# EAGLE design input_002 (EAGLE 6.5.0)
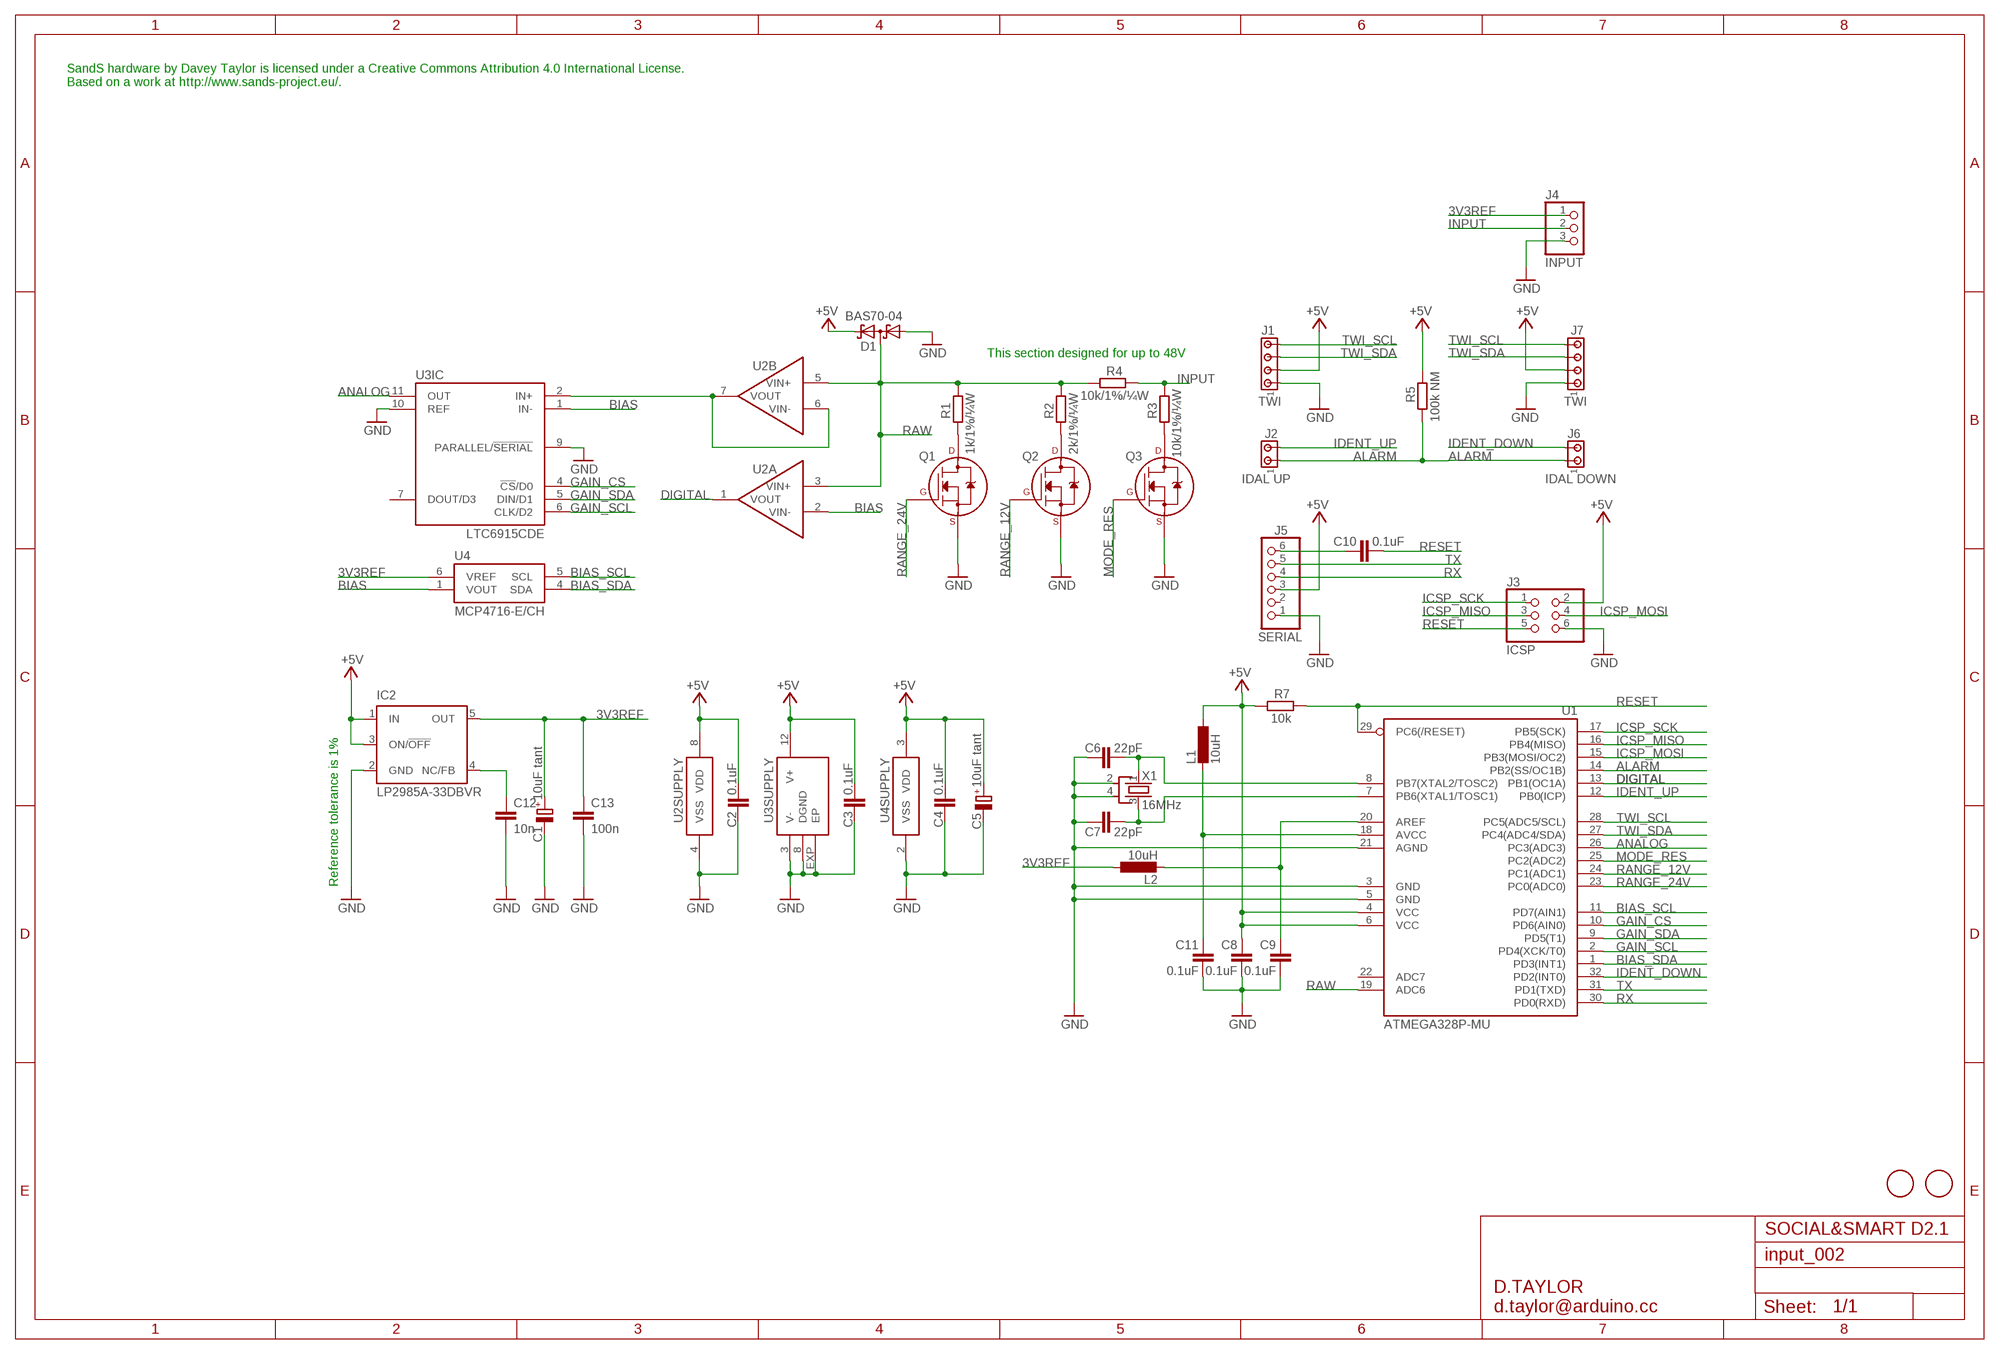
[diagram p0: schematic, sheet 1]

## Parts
C1  10uF tant  CPOL-EUSMCB  [SMC_B]
C2  0.1uF  C-EUC0603  [C0603]
C3  0.1uF  C-EUC0603  [C0603]
C4  0.1uF  C-EUC0603  [C0603]
C5  10uF tant  CPOL-EUSMCB  [SMC_B]
C6  22pF  C-EUC0603  [C0603]
C7  22pF  C-EUC0603  [C0603]
C8  0.1uF  C-EUC0603  [C0603]
C9  0.1uF  C-EUC0603  [C0603]
C10  0.1uF  C-EUC0603  [C0603]
C11  0.1uF  C-EUC0603  [C0603]
C12  10n  C-EUC0603  [C0603-ROUND]
C13  100n  C-EUC0603  [C0603-ROUND]
D1  BAS70-04  [SOT23]
IC2  LP2985A-33DBVR  LP2985-XXDBVR33  [SOT23-DBV]
J1  TWI  MTA04-100  [10X04MTA]
J2  IDAL UP  MTA02-100  [10X02MTA]
J3  ICSP  PINHD-2X3  [2X03]
J4  INPUT  MKDS_1,5/3-5,08  [MKDS1,5/3-5,08]
J5  SERIAL  PINHD-1X6  [1X06]
J6  IDAL DOWN  MTA02-100  [10X02MTA]
J7  TWI  MTA04-100  [10X04MTA]
L1  10uH  L-EUL2012C  [L2012C]
L2  10uH  L-EUL2012C  [L2012C]
Q1  2N7002_SOT23  [SOT-23]
Q2  2N7002_SOT23  [SOT-23]
Q3  2N7002_SOT23  [SOT-23]
R1  1k/1%/¼W  R-EU_R1206  [R1206]
R2  2k/1%/¼W  R-EU_R1206  [R1206]
R3  10k/1%/¼W  R-EU_R1206  [R1206]
R4  10k/1%/¼W  R-EU_R1206  [R1206]
R5  100k NM  R-EU_R0603  [R0603]
R7  10k  R-EU_R0603  [R0603]
U1  ATMEGA328P-MU  [MLF32-M1-A]
U2  MCP6402-E/SN  [SO8]
U3  LTC6915CDE  [DFN12]
U4  MCP4716-E/CH  [SOT-23-6]
U$5  FIDUCIALMOUNT  [FIDUCIA-MOUNT]
U$6  FIDUCIALMOUNT  [FIDUCIA-MOUNT]
X1  16MHz  CRYSTAL-KX7  [XTAL-3.2-2.5]

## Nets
3V3REF: C1.+ C13.1 IC2.5(OUT) J4.1 L2.1 U4.6(VREF)
+5V: C2.1 C3.1 C4.1 C5.+ C8.1 D1.2(C2) IC2.1(IN) IC2.3(ON/!OFF) J1.2 J3.2 J5.3 J7.2 L1.1 R5.2 R7.1 U1.4(VCC) U1.6(VCC) U2.8(SUPPLY:VDD) U3.12(SUPPLY:V+) U4.3(VDD)
ALARM: J2.1 J6.1 R5.1 U1.14(PB2(SS/OC1B))
ANALOG: U1.26(PC3(ADC3)) U3.11(IC:OUT)
BIAS: U2.2(A:VIN-) U3.1(IC:IN-) U4.1(VOUT)
BIAS_SCL: U1.11(PD7(AIN1)) U4.5(SCL)
BIAS_SDA: U1.1(PD3(INT1)) U4.4(SDA)
DIGITAL: U1.13(PB1(OC1A)) U2.1(A:VOUT)
GAIN_CS: U1.10(PD6(AIN0)) U3.4(IC:!CS!/D0)
GAIN_SCL: U1.2(PD4(XCK/T0)) U3.6(IC:CLK/D2)
GAIN_SDA: U1.9(PD5(T1)) U3.5(IC:DIN/D1)
GND: C1.- C2.2 C3.2 C4.2 C5.- C6.1 C7.1 C8.2 C9.2 C11.2 C12.2 C13.2 D1.1(A1) IC2.2(GND) J1.1 J3.6 J4.3 J5.1 J7.1 Q1.2(S) Q2.2(S) Q3.2(S) U1.3(GND) U1.5(GND) U1.21(AGND) U2.4(SUPPLY:VSS) U3.3(SUPPLY:V-) U3.8(SUPPLY:DGND) U3.9(IC:PARALLEL/!SERIAL) U3.10(IC:REF) U3.EXP(SUPPLY:EP) U4.2(VSS) X1.2(SH1) X1.4(SH2)
ICSP_MISO: J3.3 U1.16(PB4(MISO))
ICSP_MOSI: J3.4 U1.15(PB3(MOSI/OC2))
ICSP_SCK: J3.1 U1.17(PB5(SCK))
IDENT_DOWN: J6.2 U1.32(PD2(INT0))
IDENT_UP: J2.2 U1.12(PB0(ICP))
INPUT: J4.2 R3.2 R4.2
MODE_RES: Q3.1(G) U1.25(PC2(ADC2))
N$1: Q1.3(D) R1.1
N$2: Q2.3(D) R2.1
N$3: Q3.3(D) R3.1
N$4: C12.1 IC2.4(NC/FB)
N$5: U2.6(B:VIN-) U2.7(B:VOUT) U3.2(IC:IN+)
N$6: C6.2 U1.8(PB7(XTAL2/TOSC2)) X1.1(X1)
N$7: C7.2 U1.7(PB6(XTAL1/TOSC1)) X1.3(X2)
N$8: C11.1 L1.2 U1.18(AVCC)
N$9: C10.1 J5.6
N$10: C9.1 L2.2 U1.20(AREF)
RANGE_12V: Q2.1(G) U1.24(PC1(ADC1))
RANGE_24V: Q1.1(G) U1.23(PC0(ADC0))
RAW: D1.3(C1A2) R1.2 R2.2 R4.1 U1.19(ADC6) U2.3(A:VIN+) U2.5(B:VIN+)
RESET: C10.2 J3.5 R7.2 U1.29(PC6(/RESET))
RX: J5.4 U1.30(PD0(RXD))
TWI_SCL: J1.4 J7.4 U1.28(PC5(ADC5/SCL))
TWI_SDA: J1.3 J7.3 U1.27(PC4(ADC4/SDA))
TX: J5.5 U1.31(PD1(TXD))
Unconnected: J5.2 U1.22(ADC7) U3.7(IC:DOUT/D3)

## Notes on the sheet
- SandS hardware by Davey Taylor is licensed under a Creative Commons Attribution 4.0 International License.
  Based on a work at http://www.sands-project.eu/.
- This section designed for up to 48V
- Reference tolerance is 1%
- SOCIAL&SMART D2.1
- D.TAYLOR
  d.taylor@arduino.cc

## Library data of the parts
C1 C5 = rcl:CPOL-EU: POLARIZED CAPACITOR, European symbol
C2-C4 C6-C11 = rcl:C-EU: CAPACITOR, European symbol
C12 C13 = SmartPrj:C-EU: CAPACITOR, European symbol
D1 = diode:BAS70-04: Silicon Schottky Diodes General-purpose diode for high-speed switching
IC2 = SmartPrj:LP2985-XXDBVR: ULTRALOW-POWER 50-mA LOW-DROPOUT LINEAR REGULATORS 50-mA Low-Dropout Regulator Source: http://focus.ti.com/lit/ds/symlink/tps77001.pdf
J1 J7 = d_taylor:MTA04-100: AMP connector
J2 J6 = d_taylor:MTA02-100: AMP connector
J3 = pinhead:PINHD-2X3: PIN HEADER
J4 = d_taylor:MKDS_1,5/3-5,08: MKDSN 1,5/ 3-5,08 Printklemme Nennstrom: 13,5 A Nennspannung: 250 V Rastermaß: 5,08 mm Polzahl: 3 Anschlussart: Schraubanschluss Montage: Löten Anschlussrichtung Leiter/Platine: 0 ° Artikelnummer: 1729131 Source: http://eshop.phoenixcontact.com .. 1729131.pdf; MPN: SMKDSN1,5/3-5,08; OC_FARNELL: 1792904; OC_NEWARK: 70R0299
J5 = pinhead:PINHD-1X6: PIN HEADER
L1 L2 = rcl:L-EU: INDUCTOR, European symbol
Q1-Q3 = d_taylor:2N700*: 2N7000, 2N7002, NDS7002A N-channel enhancement mode MOSFET
R1-R5 R7 = rcl:R-EU_: RESISTOR, European symbol
U1 = d_taylor:ATMEGA*: MICROCONTROLLER 8 Kbytes FLASH 1 kbytes SRAM 512 bytes EEPROM USART 6-channel 10 bit ADC 2-channel 8 bit ADC Source: avr.lbr
U2 = d_taylor:MCP6402
U3 = d_taylor:LTC6915*DE
U4 = d_taylor:MCP47*6
U$5 U$6 = SmartPrj:FIDUCIALMOUNT
X1 = d_taylor:CRYSTAL-KX7

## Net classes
1 PWR: width 0.406 mm, clearance 0.254 mm
2 gnd: width 0.203 mm, drill 0.406 mm, clearance 0.203 mm
3 usbvcc: width 0.203 mm, drill 0.406 mm, clearance 0.203 mm

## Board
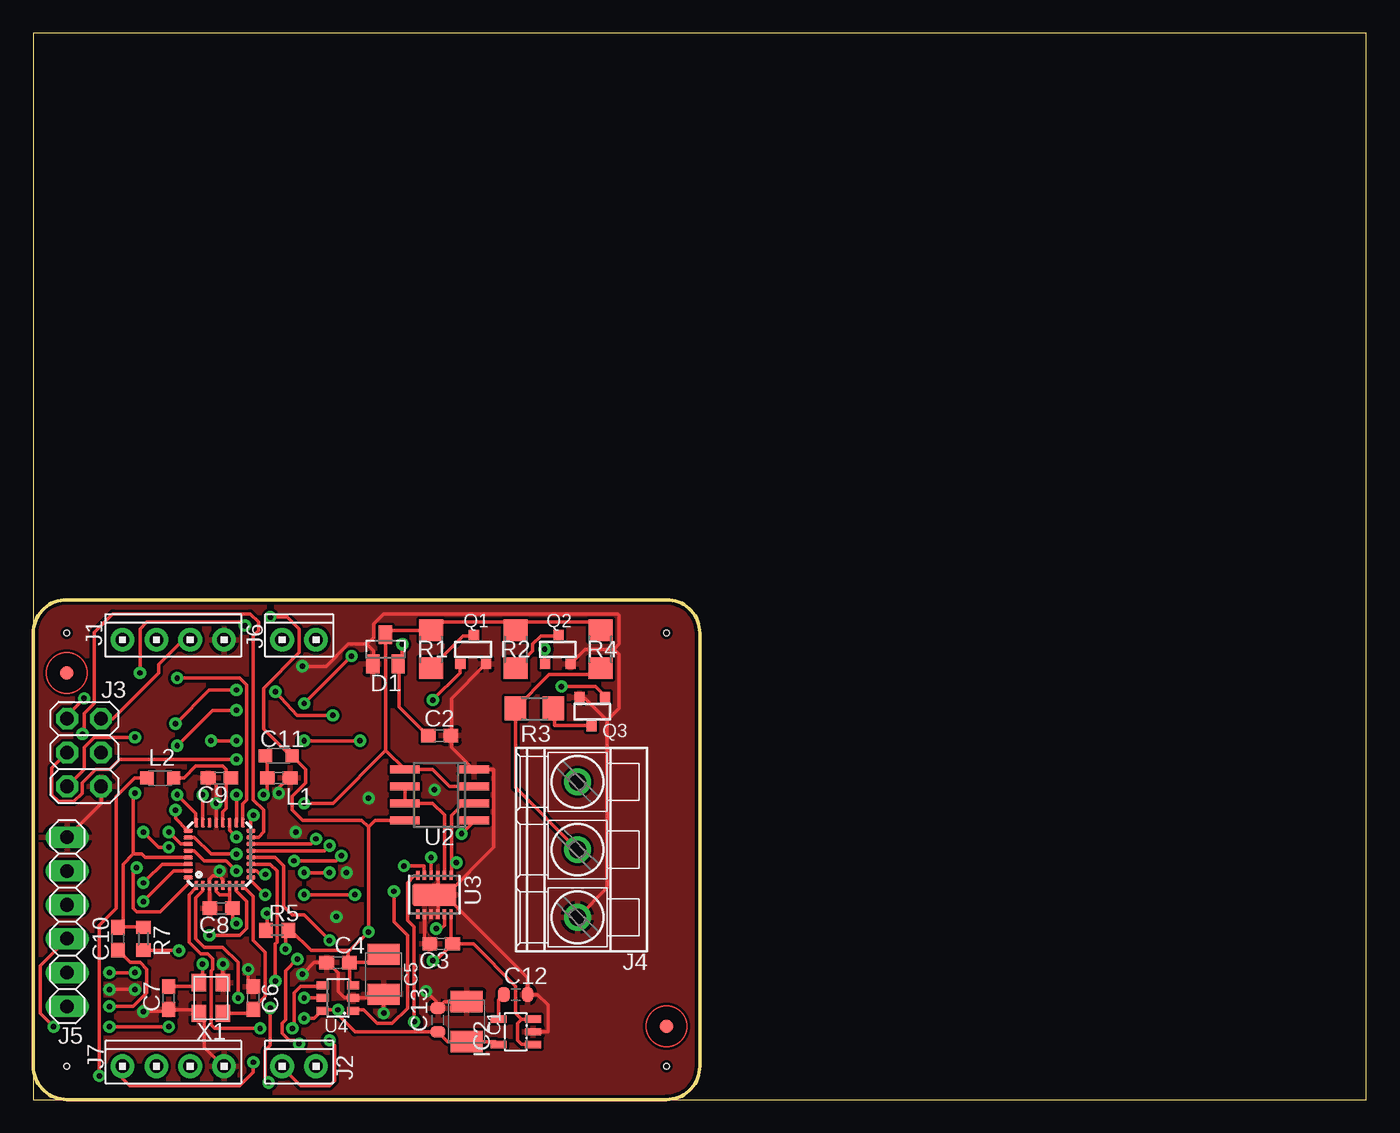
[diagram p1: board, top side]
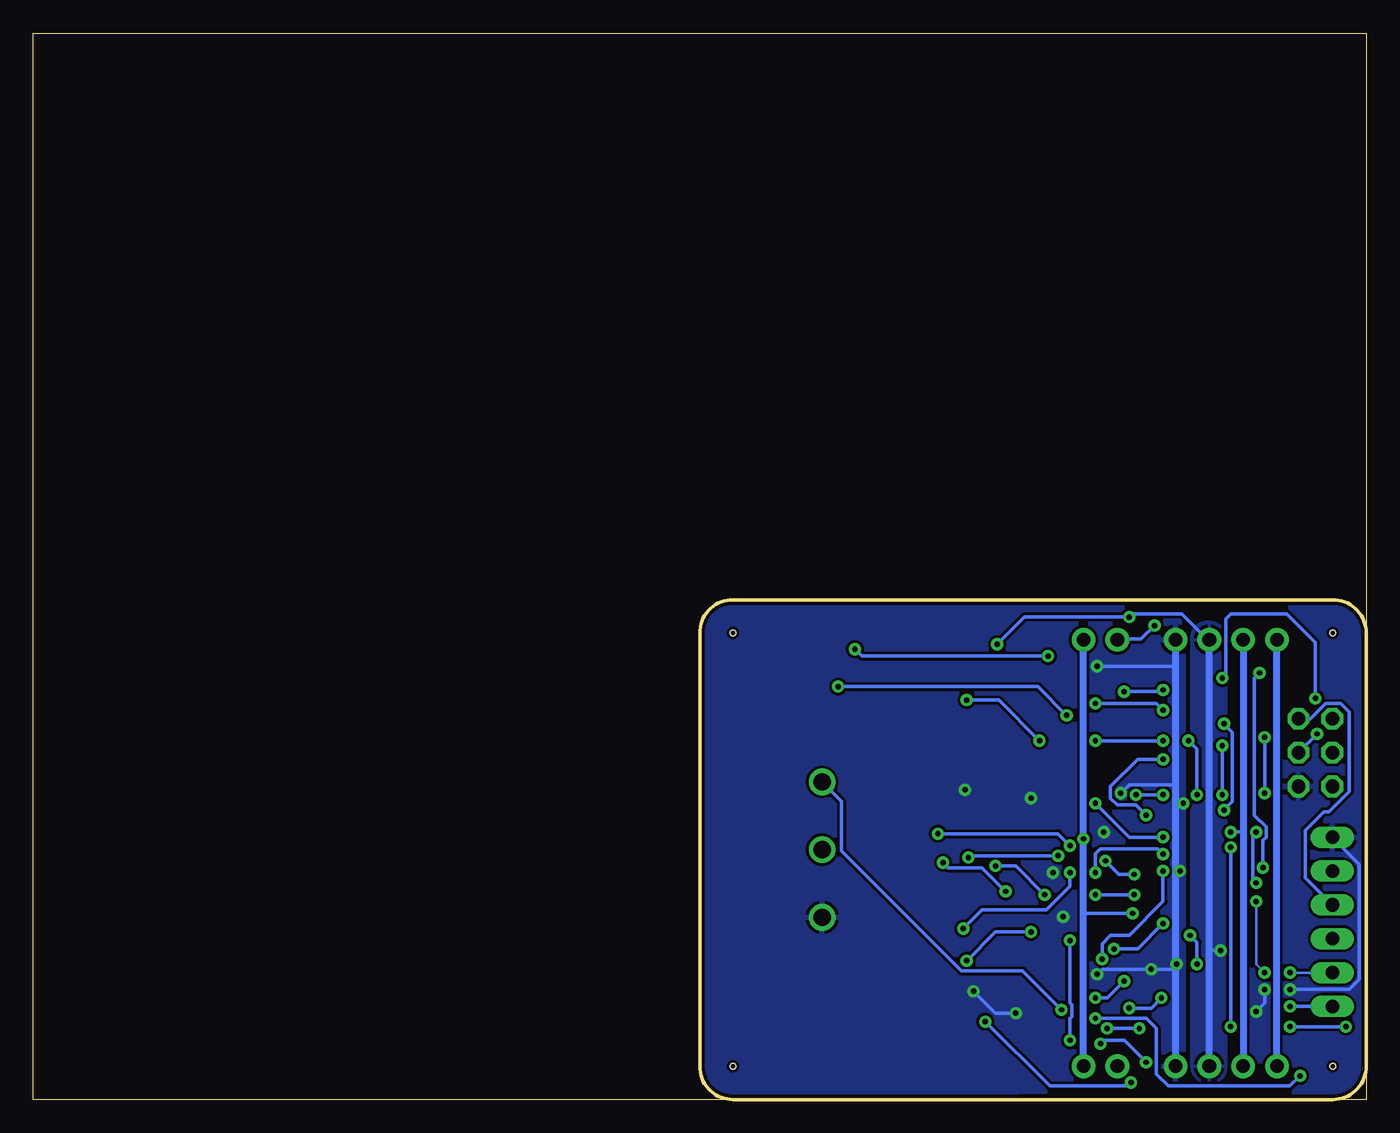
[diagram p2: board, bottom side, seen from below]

Size 100 x 80 mm. Coordinates in mm from the lower left corner, seen from the top.
Outline: 0,35 0,80 100,80 100,0 0,0 0,35
Outline: 0,35 arc-90 2.5,37.5 47.5,37.5 arc-90 50,35 50,2.5 arc-90 47.5,0 2.5,0 arc-90 0,2.5 0,35
Copper layers (1*16): Top 0.035mm / dielectric 1.5mm / Bottom 0.035mm
Design rules "smartprj-mini *": minimum track width 8mil, minimum drill 10mil, track to track 8mil, track to pad 8mil, pad to pad 0.2mm, via to via 7mil, smd to smd 4mil, copper to edge 10mil, drill to drill 8mil, minimum pad ring 12mil, minimum via ring 10mil, stop-mask expansion 2mil, vias tented up to drill 20mil, thermal gap 10mil
Holes 0.41 mm at 2.5,35 2.5,2.5 47.5,2.5 47.5,35

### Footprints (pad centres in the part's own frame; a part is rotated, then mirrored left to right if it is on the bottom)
SMC_B = smd 1.6 x 2.4: + -1.5,0; - 1.5,0
C0603 = smd 1.1 x 1: 1 -0.85,0; 2 0.85,0
C0603-ROUND = smd 0.898 x 1.1: 1 -0.889,0; 2 0.889,0
SOT23 = smd 1 x 1.4: 1 -0.95,-1.1; 2 0.95,-1.1; 3 0,1.1
SOT23-DBV = smd 0.55 x 1.2: 1 -0.95,-1.3; 2 0,-1.3; 3 0.95,-1.3; 4 0.95,1.3; 5 -0.95,1.3
10X04MTA = drill 1.016 pad 1.778: 1 3.81,0; 2 1.27,0; 3 -1.27,0; 4 -3.81,0
10X02MTA = drill 1.016 pad 1.778: 1 1.27,0; 2 -1.27,0
2X03 = drill 1.016 octagon: 1 -2.54,-1.27; 2 -2.54,1.27; 3 0,-1.27; 4 0,1.27; 5 2.54,-1.27; 6 2.54,1.27
MKDS1,5/3-5,08 = drill 1.3 pad 2: 1 -5.08,0; 2 0,0; 3 5.08,0
1X06 = drill 1.016 long: 1 -6.35,0; 2 -3.81,0; 3 -1.27,0; 4 1.27,0; 5 3.81,0; 6 6.35,0
L2012C = smd 1 x 1: 1 -1,0; 2 1,0
SOT-23 = smd 0.762 x 0.762: 1 -0.979,-1.101; 2 0.94,-1.101; 3 0.025,1.067
R1206 = smd 1.6 x 1.803: 1 -1.422,0; 2 1.422,0
R0603 = smd 1 x 1.1: 1 -0.85,0; 2 0.85,0
MLF32-M1-A = smd 0.7 x 0.3: 1 -2.35,1.75; 2 -2.35,1.25; 3 -2.35,0.75; 4 -2.35,0.25; 5 -2.35,-0.25; 6 -2.35,-0.75; 7 -2.35,-1.25; 8 -2.35,-1.75; 17 2.35,-1.75; 18 2.35,-1.25; 19 2.35,-0.75; 20 2.35,-0.25; 21 2.35,0.25; 22 2.35,0.75; 23 2.35,1.25; 24 2.35,1.75 | smd 0.3 x 0.7: 9 -1.75,-2.35; 10 -1.25,-2.35; 11 -0.75,-2.35; 12 -0.25,-2.35; 13 0.25,-2.35; 14 0.75,-2.35; 15 1.25,-2.35; 16 1.75,-2.35; 25 1.75,2.35; 26 1.25,2.35; 27 0.75,2.35; 28 0.25,2.35; 29 -0.25,2.35; 30 -0.75,2.35; 31 -1.25,2.35; 32 -1.75,2.35
SO8 = smd 0.6 x 2.2: 1 -1.905,-2.6; 2 -0.635,-2.6; 3 0.635,-2.6; 4 1.905,-2.6; 5 1.905,2.6; 6 0.635,2.6; 7 -0.635,2.6; 8 -1.905,2.6
DFN12 = smd 0.25 x 0.7: 1 -1.25,-1.45; 2 -0.75,-1.45; 3 -0.25,-1.45; 4 0.25,-1.45; 5 0.75,-1.45; 6 1.25,-1.45; 7 1.25,1.45; 8 0.75,1.45; 9 0.25,1.45; 10 -0.25,1.45; 11 -0.75,1.45; 12 -1.25,1.45 | smd 3.3 x 1.7: EXP 0,0
SOT-23-6 = smd 0.6 x 0.9: 1 -0.95,-1.15; 2 0,-1.15; 3 0.95,-1.15; 4 0.95,1.15; 5 0,1.15; 6 -0.95,1.15
FIDUCIA-MOUNT = smd 1.016 x 1.016: P$1 0,0
XTAL-3.2-2.5 = smd 1.3 x 1.1: 1 -1.15,-0.9; 2 1.15,-0.9; 3 1.15,0.9; 4 -1.15,0.9

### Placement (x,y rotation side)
C1  32.51,5.84 90 top
C2  30.48,27.3 0 top
C3  30.61,11.68 180 top
C4  22.86,10.29 180 top
C5  26.29,9.4 270 top
C6  16.51,7.62 270 top
C7  10.16,7.62 90 top
C8  14.1,14.35 180 top
C9  13.97,24.13 180 top
C10  6.35,12.06 90 top
C11  18.41,24.13 0 top
C12  36.2,7.87 0 top
C13  30.35,5.97 90 top
D1  26.42,33.78 0 top
IC2  36.2,5.08 90 top
J1  10.5,34.5 0 top
J2  19.94,2.5 0 top
J3  3.81,26.04 270 top
J4  40.83,18.75 270 top
J5  2.54,13.34 270 top
J6  19.94,34.5 0 top
J7  10.5,2.5 0 top
L1  18.41,25.78 180 top
L2  9.53,24.13 0 top
Q1  33.02,33.78 0 top
Q2  39.37,33.78 0 top
Q3  41.91,29.08 180 top
R1  29.84,33.78 90 top
R2  36.2,33.78 90 top
R3  37.59,29.34 180 top
R4  42.55,33.78 270 top
R5  18.29,12.7 0 top
R7  8.26,12.06 90 top
U1  13.97,18.41 90 top
U2  30.48,22.86 90 top
U3  30.1,15.37 180 top
U4  22.86,7.62 90 top
U$5  2.5,32 0 top
U$6  47.5,5.5 0 top
X1  13.34,7.62 90 top

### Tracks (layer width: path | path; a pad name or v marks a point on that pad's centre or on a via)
3V3REF  (via drill 0.41 pad 0.61)
  Top 0.254: v4.95,1.78 4.95,13.08 6.22,14.35 6.22,22.73 7.62,24.13 8.51,24.13 L2.1 | v20.32,6.1 21.08,6.1 21.59,6.6 U4.6 21.72,6.73 v22.86,6.73 22.86,6.35 24.13,5.08 C13.1 31.09,4.34 C1.+ 34.68,4.34 IC2.5 | 40.89,23.75 J4.1
  Bottom 0.254: v22.86,6.73 25.78,9.65 30.35,9.65 39.37,18.67 39.37,22.35 40.77,23.75 J4.1 | v4.95,1.78 5.71,1.02 14.86,1.02 15.75,1.91 15.75,5.33 16.51,6.1 16.64,6.1 v20.32,6.1
+5V  (via drill 0.41 pad 0.61)
  Top 0.254: 31.11,11.68 C3.1 | 25.15,20.45 25.65,20.95 27.81,20.95 U2.8 | 25.15,20.45 24.64,20.95 24.26,20.95 20.19,20.95 19.43,21.72 19.43,22.73 20.45,23.75 20.45,24.77 19.43,25.78 L1.1 19.3,25.78 17.27,27.81 17.27,30.86 19.94,33.53 19.94,35.31 19.05,36.2 v17.78,36.2 | 14.73,15.37 13.97,15.37 13.72,15.62 13.72,16 U1.4 | 14.73,15.37 14.73,16 U1.6 | 14.73,15.37 14.73,14.35 C8.1 14.95,13.5 v15.24,13.21 | U4.3 24,8.64 23.75,8.89 23.75,10.29 C4.1 | 23.62,11.18 20.83,11.18 19.3,12.7 R5.2 18.92,12.32 v18.92,11.3 | 23.62,11.18 23.62,10.29 C4.1 | 25.15,20.45 v25.15,12.57 23.75,11.18 23.62,11.18 | C2.1 29.59,27.3 27.43,29.46 27.43,32.64 D1.2 27.43,32.77 27.69,33.02 v27.69,34.16 | v10.92,11.18 8.26,11.18 R7.1 | J3.2 5.97,28.57 9.4,32 9.4,32.64 11.18,34.42 J1.2 | v29.97,10.41 30.23,10.45 C3.1 | U3.12 31.35,12.08 C3.1 | IC2.3 36.64,6.03 | 36.64,6.03 36.32,5.71 36.32,4.45 36.64,4.13 IC2.1 | C5.+ 25.68,10.29 C4.1 | 36.64,6.03 36.2,6.48 36.2,8.51 33.02,11.68 C3.1
  Bottom 0.254: v18.92,11.3 17.14,11.3 v15.24,13.21 | v29.97,10.41 27.81,12.57 v25.15,12.57 | v10.92,11.18 11.68,11.18 11.77,11.18 | J5.3 4.57,16.64 4.57,20.19 3.3,21.46 3.17,21.59 2.79,21.59 1.27,23.11 1.27,29.08 1.91,29.72 3.05,29.72 4.19,28.57 J3.2 | v27.69,34.16 25.65,36.2 v17.78,36.2 17.53,36.45 13.84,36.45 11.94,34.54 J1.2
  Bottom 0.508: J7.2 11.77,11.18 J1.2
  pour Bottom: 13.08,34.67 arc90 11.94,35.81 11.81,35.81 arc90 10.54,34.54 10.54,2.54 10.54,2.41 arc90 11.68,1.27 11.81,1.27 arc90 13.08,2.54
ALARM  (via drill 0.41 pad 0.61)
  Top 0.254: v21.21,19.56 20.83,19.18 16.38,19.18 U1.14 | v17.53,13.97 17.53,12.7 R5.1
  Bottom 0.254: 21.21,13.97 v17.53,13.97
  Bottom 0.508: J2.1 21.21,13.97 v21.21,19.56 J6.1
ANALOG  (via drill 0.41 pad 0.61)
  Top 0.254: v20.32,17.02 v22.23,17.02 | v15.24,18.41 13.34,18.41 12.09,19.66 U1.26 | U3.11 30.85,13.07 30.61,12.83 v30.23,12.83
  Bottom 0.254: v30.23,12.83 28.83,14.22 24,14.22 22.23,16 v22.23,17.02 | v20.32,17.02 20.32,18.41 19.94,18.8 15.62,18.8 v15.24,18.41
BIAS  (via drill 0.41 pad 0.61)
  Top 0.254: 31.37,17.78 31.37,21.34 32.26,22.23 33.02,22.23 U2.2 | 31.37,17.78 31.37,16.89 U3.1 | v27.05,15.62 27.05,13.34 28.07,12.32 28.07,6.86 26.92,5.71 25.78,5.71 24.77,6.73 24.13,6.73 U4.1 | 31.37,17.78 v31.75,17.78
  Bottom 0.254: v27.05,15.62 28.83,17.4 31.37,17.4 v31.75,17.78
BIAS_SCL  (via drill 0.41 pad 0.61)
  Top 0.254: v18.16,8.89 18.16,11.68 18.29,11.81 18.29,13.34 18.29,13.59 18.29,17.14 17.78,17.65 16.38,17.65 U1.11 | v20.32,7.62 21.59,7.62 U4.5
  Bottom 0.254: v18.16,8.89 19.43,7.62 v20.32,7.62
BIAS_SDA  (via drill 0.41 pad 0.61)
  Top 0.254: v17.02,5.33 13.59,5.33 13.34,5.59 13.34,9.65 13.46,9.78 13.46,10.54 13.08,10.92 12.57,10.92 11.68,11.81 11.68,15.37 12.19,15.88 12.22,16.03 U1.1 | v19.43,5.33 19.56,5.46 19.56,8 20.07,8.51 21.59,8.51 U4.4
  Bottom 0.254: v19.43,5.33 v17.02,5.33
DIGITAL  (via drill 0.41 pad 0.61)
  Top 0.254: v22.23,19.05 21.84,18.67 16.38,18.67 U1.13 | v32.13,19.94 33.02,20.83 33.02,20.95 U2.1
  Bottom 0.254: v22.23,19.05 23.11,19.94 v32.13,19.94
GAIN_CS  (via drill 0.41 pad 0.61)
  Top 0.254: v29.84,18.16 29.84,16.89 U3.4 | v23.11,18.29 22.73,17.91 v19.56,17.91 | v17.4,16.89 17.02,16.89 16.76,17.14 16.38,17.14 U1.10
  Bottom 0.254: v29.84,18.16 29.72,18.29 v23.11,18.29 | v19.56,17.91 18.54,16.89 v17.4,16.89
GAIN_SCL  (via drill 0.41 pad 0.61)
  Top 0.254: v15.37,7.62 15.37,10.29 14.22,11.43 12.83,11.43 12.19,12.06 12.19,15.11 12.72,15.64 U1.2 | v17.78,6.86 17.78,4.06 17.4,3.68 17.4,1.52 v17.65,1.27 | v28.57,5.84 28.57,9.53 28.57,9.78 28.57,12.95 28.07,13.46 28.07,16.26 28.57,16.76 28.83,16.76 U3.6
  Bottom 0.254: v15.37,7.62 16.13,6.86 v17.78,6.86 | v17.65,1.27 17.91,1.02 23.75,1.02 v28.57,5.84
GAIN_SDA  (via drill 0.41 pad 0.61)
  Top 0.254: v17.4,15.37 16.38,16.38 16.38,16.64 U1.9 | v24.13,15.37 v20.32,15.37 | v27.81,17.53 29.34,17.53 29.34,16.89 U3.5
  Bottom 0.254: v20.32,15.37 v17.4,15.37 | v24.13,15.37 26.29,17.53 v27.81,17.53
GND  (via drill 0.41, 0.41 pad 0.61)
  Top 0.203: 29.72,11.81 C3.2 | 31.37,27.3 C2.2 | 30.35,15.37 U3.EXP
  Top 0.254: J5.1 5.08,22.23 J3.6 | 13.21,14.48 C8.2 13.22,14.45 U1.3 13.21,16.13 13.21,16.51 13.46,16.76 13.97,16.76 | 13.97,16.76 14.22,16.51 14.22,16.13 U1.5 | U1.21 13.72,20.83 v13.72,22.23 13.72,23.62 13.21,24.13 C9.2 | v16.13,9.78 16.13,8.89 16.51,8.51 C6.1 | v18.41,22.99 18.41,23.37 19.18,24.13 C11.2 | v14.22,10.16 14.22,8.89 X1.2 | J7.1 14.22,2.54 12.83,3.94 12.83,5.97 12.45,6.35 X1.4 12.32,6.48 12.32,6.73 10.16,6.73 C7.1 10.16,6.6 v8.26,6.6 | v13.97,17.14 13.97,16.76 | v20.19,9.4 21.08,10.29 21.97,10.29 C4.2 22.1,10.29 22.86,9.53 22.86,8.13 23.37,7.62 U4.2 26.01,7.62 C5.- v26.29,6.48 | v7.62,8.26 v5.71,8.26 | 30.35,15.37 30.35,15.88 | 30.35,15.88 30.35,16.76 U3.3 | 29.72,11.81 C3.2 29.35,11.78 U3.8 U3.9 U3.10 30.35,13.97 30.35,15.11 U3.EXP | 31.37,27.3 31.37,30.1 33.91,32.64 Q1.2 | 31.37,27.3 31.37,26.42 33.02,24.77 U2.4 33.15,24.77 34.54,24.77 34.54,18.92 30.99,15.37 30.35,15.37 | 31.37,27.3 C2.2 | 30.35,15.88 32.77,13.46 37.08,9.14 C12.2 37.85,7.87 38.61,7.11 38.61,5.08 IC2.2 | 30.35,15.88 U3.EXP | 30.35,15.37 U3.EXP | 43.05,28.45 43.94,29.34 43.94,32.77 43.94,33.4 43.56,33.78 | 43.05,28.45 41.4,30.1 41.02,30.1 Q3.2 | Q2.2 40.39,32.77 41.4,33.78 43.43,33.78 43.56,33.78 | 25.02,34.16 25.53,34.67 25.53,35.69 26.29,36.45 43.81,36.45 43.94,36.32 43.94,34.16 43.56,33.78 | 25.02,34.16 25.53,33.66 25.53,32.77 D1.1 | 43.05,28.45 43.05,15.88 40.89,13.72 J4.3 | v20.19,32.51 21.97,32.51 23.62,34.16 25.02,34.16 | C1.- 30.84,7.34 C13.2 30.23,6.99 30.23,7.37 v29.46,8.13
  Bottom 0.254: 14.31,9.78 14.48,9.78 v16.13,9.78 19.81,9.78 v20.19,9.4 | v18.41,22.99 17.78,23.62 14.48,23.62 14.31,23.62 | v14.22,10.16 14.31,10.16 | v13.72,22.23 14.22,22.23 14.31,22.23 | v13.97,17.14 14.22,17.14 14.31,17.14 | J5.1 0.51,17.65 0.51,9.02 1.27,8.26 v5.71,8.26 | v7.62,8.26 7.62,7.24 v8.26,6.6 | v20.19,32.51 14.48,32.51 14.31,32.51 | v26.29,6.48 27.81,6.48 v29.46,8.13
  Bottom 0.508: J1.1 14.31,32.51 14.31,23.62 14.31,22.23 14.31,17.14 14.31,10.16 14.31,9.78 J7.1
  other vias: 19.68,20.07 22.73,13.72 25.15,22.61 30.1,23.24 23.5,17.02
  pour Top: 0.5,35 arc-90 2.5,37 47.5,37 arc-90 49.5,35 49.5,2.5 arc-90 47.5,0.5 2.5,0.5 arc-90 0.5,2.5
  pour Bottom: 0.5,35 arc-90 2.5,37 47.5,37 arc-90 49.5,35 49.5,2.5 arc-90 47.5,0.5 15.49,0.64 arc-90 13.72,2.41 13.72,34.42 arc90 11.81,36.45 arc90 9.91,34.54 9.91,2.54 arc-90 7.87,0.5 2.5,0.5 arc-90 0.5,2.5
ICSP_MISO  (via drill 0.41 pad 0.61)
  Top 0.254: v15.24,25.53 6.48,25.53 5.71,24.77 5.33,24.77 4.7,24.77 3.68,23.75 3.68,22.99 3.05,22.35 1.91,22.35 1.4,22.86 1.4,24.89 J3.3 | U1.16 16.32,21.15 v16.51,21.34
  Bottom 0.254: v16.51,21.34 17.27,22.1 18.67,22.1 19.18,22.61 19.18,23.5 17.14,25.53 v15.24,25.53
ICSP_MOSI  (via drill 0.41 pad 0.61)
  Top 0.254: v3.68,27.43 3.81,27.56 3.81,28.96 4.57,29.72 4.57,35.05 5.97,36.45 16.26,36.45 16.89,35.81 16.89,35.18 16.51,34.8 16.51,22.48 17.27,21.72 17.27,20.07 16.89,19.68 16.38,19.68 U1.15
  Bottom 0.254: J3.4 v3.68,27.43
ICSP_SCK  (via drill 0.41 pad 0.61)
  Top 0.254: v10.79,31.62 15.49,31.62 16,31.11 16,22.48 15.72,22.2 U1.17 | v3.81,30.1 2.54,28.83 J3.1
  Bottom 0.254: v10.79,31.62 10.54,31.88 10.54,32 10.54,35.94 10.54,36.07 10.16,36.45 5.97,36.45 3.81,34.29 v3.81,30.1
IDENT_DOWN  (via drill 0.41 pad 0.61)
  Top 0.254: v7.75,17.4 7.49,17.14 7.49,14.35 7.75,14.1 9.02,14.1 9.53,14.1 11.62,16.19 U1.32 | v8,32 8,32.77 8,35.31 8.51,35.81 15.62,35.81 v15.88,35.56
  Bottom 0.254: v7.75,17.4 7.75,19.43 7.49,19.68 7.49,20.45 8.38,21.34 8.38,31.62 v8,32 | v15.88,35.56 16.89,34.54 18.67,34.54 J6.2
IDENT_UP  (via drill 0.41 pad 0.61)
  Top 0.203: 18.67,2.41 J2.2
  Top 0.254: v22.23,11.94 20.32,13.84 19.43,13.84 18.8,14.48 18.8,17.53 18.16,18.16 16.38,18.16 U1.12 | v22.23,4.45 22.61,4.06 22.61,1.4 22.23,1.02 20.57,1.02 20.07,1.02 18.67,2.41
  Bottom 0.254: v22.23,11.94 22.23,7.24 22.1,7.11 22.1,6.22 22.23,6.1 v22.23,4.45
INPUT
  Top 0.254: J4.2 36.17,23.41 R3.2 38.71,31.88 41.4,31.88 41.94,31.88 R4.2
MODE_RES  (via drill 0.41 pad 0.61)
  Top 0.254: v10.67,21.72 10.67,21.08 11.56,20.19 U1.25 | v10.67,28.19 13.21,30.73 v15.24,30.73 | v18.16,30.61 19.81,28.83 v22.48,28.83 | v39.62,30.99 42.16,30.99 42.93,30.23 42.93,30.1 Q3.1
  Bottom 0.254: v10.67,21.72 10.03,22.35 10.03,27.56 v10.67,28.19 | v15.24,30.73 15.49,30.61 v18.16,30.61 | v22.48,28.83 24.64,30.99 39.12,30.99 v39.62,30.99
N$1
  Top 0.254: Q1.3 33.02,34.8 32.26,34.8 29.84,32.38 R1.1
N$2
  Top 0.254: Q2.3 39.37,34.8 38.1,34.8 37.47,34.16 37.47,33.66 36.2,32.38 R2.1
N$3
  Top 0.254: Q3.3 41.78,28.07 39.12,28.07 39.12,29.34 R3.1
N$4
  Top 0.254: 35.31,5.97 35.24,6.03 IC2.4 34.9,7.46 C12.1
N$5
  Top 0.254: U2.6 U2.7 29.97,22.23 30.85,21.35 U3.2
N$6
  Top 0.254: X1.1 14.35,6.48 16.51,6.48 16.51,6.73 C6.2 16.51,6.86 17.4,7.75 17.4,9.91 17.4,11.05 16.51,11.94 16.51,15.24 15.72,16.03 U1.8
N$7  (via drill 0.41, 0.41 pad 0.61)
  Top 0.254: v12.7,10.16 12.7,9.14 X1.3 12.32,8.76 12.32,8.51 10.16,8.51 C7.2 | 15.24,16.13 U1.7 15.22,15.64 16,14.86 16,12.83 15.49,12.32 13.34,12.32 v13.21,12.32
  Bottom 0.254: v12.7,10.16 12.7,11.81 v13.21,12.32
N$8  (via drill 0.41 pad 0.61)
  Top 0.203: 17.53,24.13 C11.1
  Top 0.254: v15.24,22.86 15.24,20.83 U1.18 | v17.27,22.86 17.53,23.11 17.53,24.13 | 17.53,24.13 17.53,25.78 L1.2 | 17.53,24.13 C11.1
  Bottom 0.254: v17.27,22.86 v15.24,22.86
N$9  (via drill 0.41 pad 0.61)
  Top 0.254: v5.71,6.99 5.84,6.99 7.49,6.99 8.51,8 8.51,9.78 8,10.29 7.49,10.29 7.28,10.29 C10.1 6.35,11.3
  Bottom 0.254: v5.71,6.99 5.46,6.99 J5.6
N$10
  Top 0.254: U1.20 14.22,20.83 14.22,21.59 14.48,21.84 14.48,23.88 14.73,24.13 C9.1 14.48,24 14.48,24.77 14.22,25.02 12.19,25.02 11.3,24.13 10.54,24.13 L2.2
RANGE_12V  (via drill 0.41 pad 0.61)
  Top 0.254: v10.79,22.86 11.43,22.23 12.19,21.46 12.19,20.83 U1.24 | v10.79,26.54 13.46,29.21 v15.24,29.21 | v23.88,33.27 v20.32,29.72 | v38.35,33.78 38.35,33.66 38.35,32.77 Q2.1
  Bottom 0.254: v10.79,26.54 v10.79,22.86 | v15.24,29.21 15.75,29.72 v20.32,29.72 | v23.88,33.27 37.85,33.27 v38.35,33.78
RANGE_24V  (via drill 0.41 pad 0.61)
  Top 0.254: v15.24,26.92 v13.34,26.92 | v24.51,26.92 v20.32,26.92 | v29.97,29.97 32,32 32,32.38 32,32.64 Q1.1 | U1.23 12.72,22.84 v12.7,22.86
  Bottom 0.254: v12.7,22.86 12.7,26.29 v13.34,26.92 | v15.24,26.92 15.62,26.92 v20.32,26.92 | v24.51,26.92 27.56,29.97 v29.97,29.97
RAW  (via drill 0.41)
  Top 0.254: R4.1 41.94,35.81 39.37,35.81 36.8,35.81 R2.2 35.59,35.81 33.02,35.81 30.45,35.81 R1.2 26.74,35.2 D1.3 26.42,26.23 26.45,26.2 | 26.45,26.2 U2.5 29.97,24.77 31.24,23.5 U2.3 | U1.19 14.72,20.2 v15.24,19.68 | v20.32,22.23 22.48,22.23 26.45,26.2
  Bottom 0.254: v15.24,19.68 17.78,19.68 v20.32,22.23
RESET  (via drill 0.41 pad 0.51, 0.41 pad 0.61)
  Top 0.254: 7.49,18.41 8.13,18.41 8.38,18.16 11.56,18.16 U1.29 | 7.49,18.41 6.73,17.65 6.73,13.34 6.35,12.95 C10.2 6.48,12.95 8.26,12.95 R7.2 | J3.5 3.56,24.51 3.81,24.77 3.81,26.42 4.57,27.18 v7.62,27.18 | v7.62,22.99 7.49,22.86 7.49,18.41
  Bottom 0.254: v7.62,22.99 v7.62,27.18
RX  (via drill 0.41 pad 0.61)
  Top 0.254: v8.26,16.26 8.51,16.51 9.65,17.65 11.56,17.65 U1.30 | v8.26,20.07 9.4,18.92 v10.16,18.92 | v5.71,5.46 v10.16,5.46 | v1.52,5.46 0.51,6.48 0.51,10.03 J5.4
  Bottom 0.254: v8.26,16.26 8.51,16.51 8.51,19.81 v8.26,20.07 | v10.16,5.46 v10.16,18.92 | v1.52,5.46 v5.71,5.46
TWI_SCL  (via drill 0.41 pad 0.61)
  Top 0.254: v15.24,17.14 14.67,17.72 | 14.67,17.72 14.48,17.91 | v19.81,10.54 18.92,9.65 18.92,5.97 18.67,5.71 18.67,4.95 19.18,4.45 19.68,4.45 v19.94,4.19 | v16.51,2.79 16.51,2.03 15.49,1.02 7.24,1.02 6.69,1.56 J7.4 | U1.28 11.68,18.67 12.06,18.67 12.83,17.91 14.48,17.91 | 14.48,17.91 14.67,17.72
  Bottom 0.254: v15.24,17.14 15.24,14.86 17.78,12.32 18.03,12.32 19.18,12.32 19.81,11.68 v19.81,10.54 | v19.94,4.19 19.68,4.45 18.16,4.45 v16.51,2.79
  Bottom 0.508: J7.4 J1.4
TWI_SDA  (via drill 0.41 pad 0.61)
  Top 0.254: U1.27 11.06,19.16 v10.16,20.07
  Bottom 0.254: v10.16,20.07 9.4,20.07 9.23,20.07
  Bottom 0.508: J1.3 9.23,20.07 J7.3
TX  (via drill 0.41 pad 0.61)
  Top 0.254: v8.26,14.86 10.54,17.14 11.56,17.14 U1.31 | v5.71,9.53 v7.62,9.53
  Bottom 0.203: v8.26,14.86 8.26,10.16 v7.62,9.53 | v5.71,9.53 5.33,9.53 J5.5

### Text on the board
tDocu: TWI | IDAL-D | ICSP | RREF | INPUT | SERIAL | GND | TWI | IDAL-U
